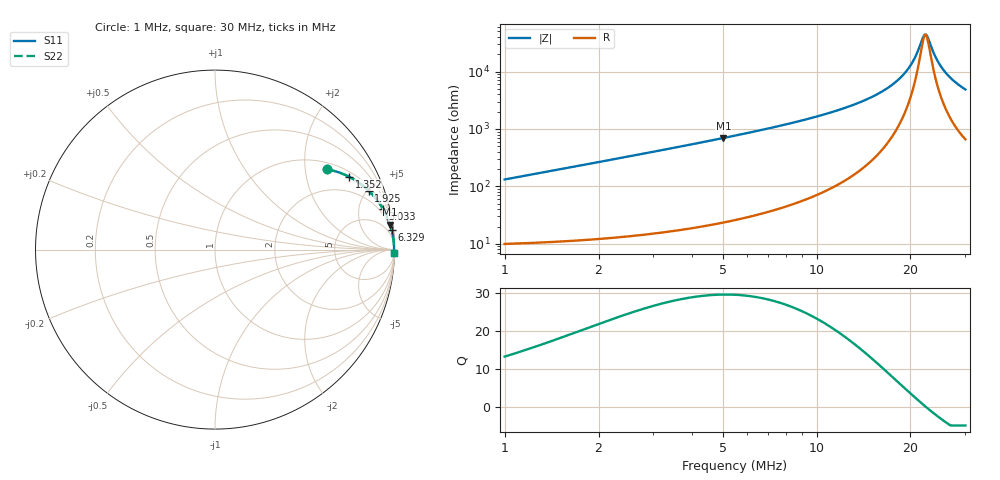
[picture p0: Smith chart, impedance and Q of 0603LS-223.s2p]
# MHz S MA R 50
!Freq  MagS11  AngS11  MagS21  AngS21  MagS12  AngS12  MagS22  AngS22
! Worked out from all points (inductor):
!   801 points, 1 MHz to 30 MHz, reference 50 ohm
!   read as one part in series: L = 20.9 uH near 1.017 MHz
!   highest Q = 29.6 at 5.031 MHz (marker M1), where L = 22 uH
!   self-resonance near 22.28 MHz
!   S11 on the Smith chart (normalised r, x): 1 MHz: 1.20, +2.63; 1.352 MHz: 1.21, +3.56; 1.925 MHz: 1.24, +5.09; 3.033 MHz: 1.30, +8.11; 6.329 MHz: 2, +18; 30 MHz: 14, -96
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1  0.7695 35.6  0.5832 -50.1  0.5832 -50.1  0.7695 35.6
1.352367  0.8511 28.4  0.4767 -58.2  0.4767 -58.2  0.8511 28.4
1.924624  0.9164 21.0  0.3596 -66.3  0.3596 -66.3  0.9164 21.0
3.033268  0.9627 13.7  0.2371 -74.2  0.2371 -74.2  0.9627 13.7
5.030748  0.9852 8.1  0.1415 -79.9  0.1415 -79.9  0.9852 8.1
5.8379  0.9887 6.9  0.1201 -81.2  0.1201 -81.2  0.9887 6.9
6.329046  0.9902 6.3  0.1096 -81.7  0.1096 -81.7  0.9902 6.3
10.67691  0.996 3.1  0.05484 -84.2  0.05484 -84.2  0.996 3.1
15.52133  0.9975 1.4  0.02539 -83.7  0.02539 -83.7  0.9975 1.4
18.39861  0.9978 0.8  0.01345 -80.0  0.01345 -80.0  0.9978 0.8
19.44412  0.9978 0.5  0.00971 -76.6  0.00971 -76.6  0.9978 0.5
20.37505  0.9978 0.4  0.006636 -70.4  0.006636 -70.4  0.9978 0.4
20.99054  0.9978 0.2  0.004776 -62.2  0.004776 -62.2  0.9978 0.2
21.90219  0.9978 0.1  0.002613 -30.9  0.002613 -30.9  0.9978 0.1
22.18333  0.9977 0.0  0.002302 -11.9  0.002302 -11.9  0.9977 0.0
22.37276  0.9977 -0.0  0.002262 2.5  0.002262 2.5  0.9977 -0.0
22.75648  0.9977 -0.1  0.002601 28.8  0.002601 28.8  0.9977 -0.1
24.15209  0.9976 -0.3  0.005802 65.8  0.005802 65.8  0.9976 -0.3
25.20106  0.9976 -0.5  0.008553 73.2  0.008553 73.2  0.9976 -0.5
26.18402  0.9975 -0.6  0.01111 76.5  0.01111 76.5  0.9975 -0.6
27.32124  0.9973 -0.8  0.014 78.7  0.014 78.7  0.9973 -0.8
30  0.997 -1.2  0.02049 81.1  0.02049 81.1  0.997 -1.2
